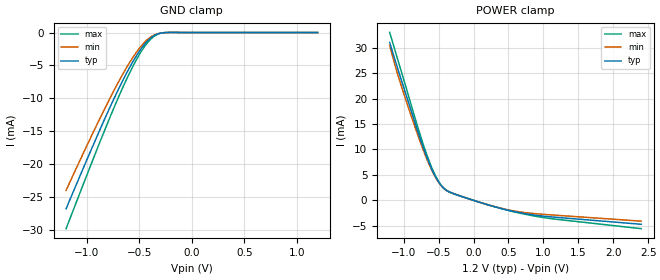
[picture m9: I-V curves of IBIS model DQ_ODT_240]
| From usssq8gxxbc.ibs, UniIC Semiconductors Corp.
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|   Model DQ_ODT_240
[Model] DQ_ODT_240
Model_type Input
Polarity   Non-Inverting
Enable   Active-High
Vinl =  8.300E-01
Vinh =  9.700E-01
C_comp   7.239E-13   7.192E-13   7.296E-13
C_comp_power_clamp   3.264E-13   3.258E-13   3.274E-13
C_comp_gnd_clamp   3.818E-13   3.778E-13   3.867E-13
[Model Spec]
Vinh   9.700E-01   9.250E-01   1.015E+00
Vinl   8.300E-01   7.850E-01   8.750E-01
[Temperature Range]   4.500E+01   9.500E+01   0.000E+00
[Voltage Range]   1.200E+00   1.140E+00   1.260E+00
[C Comp Corner]
C_comp_power_clamp   3.264E-13   3.258E-13   3.274E-13
C_comp_gnd_clamp   3.818E-13   3.778E-13   3.867E-13
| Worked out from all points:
|   GND clamp passes 1 mA (typ) near -0.40 V on its own axis
|   POWER clamp passes 1 mA (typ) near -0.22 V on its own axis
[GND_clamp]
|Voltage   I(typ)   I(min)   I(max)
-1.2V     -26.81mA   -24.01mA   -29.84mA
-875mV    -14.7mA    -12.99mA   -16.56mA
-750mV    -10.29mA   -9.021mA   -11.7mA
-650mV    -7.008mA   -6.079mA   -8.044mA
-575mV    -4.774mA   -4.091mA   -5.536mA
-500mV    -2.835mA   -2.385mA   -3.33mA
-425mV    -1.319mA   -1.082mA   -1.582mA
-375mV    -622.4uA   -504.7uA   -758.9uA
-300mV    -102.1uA   -91.47uA   -113.7uA
-225mV    4.519uA    -1.853uA   16.46uA
1.2V      0A         0A         0A
[POWER_clamp]
|Voltage   I(typ)   I(min)   I(max)
-1.2V     31.04mA    30.46mA    33mA
-1.125V   27.64mA    26.66mA    29.54mA
-1.025V   23.31mA    22.12mA    24.94mA
-825mV    14.7mA     13.92mA    15.64mA
-700mV    9.668mA    9.216mA    10.22mA
-550mV    4.819mA    4.666mA    4.977mA
-475mV    3.142mA    3.088mA    3.177mA
-400mV    2.091mA    2.102mA    2.055mA
100mV     -435.3uA   -432.3uA   -429.4uA
625mV     -2.325mA   -2.185mA   -2.396mA
1.1V      -3.233mA   -2.845mA   -3.573mA
2.4V      -4.699mA   -4.09mA    -5.562mA
